FUNCTION_BLOCK Reset_Driver_Fault_AC_Drives_DUT

VAR_IN_OUT
    SD_SMD_IO: DUT_AMCI_Stepper;
END_VAR	

VAR_INPUT
			
END_VAR

VAR_OUTPUT

END_VAR

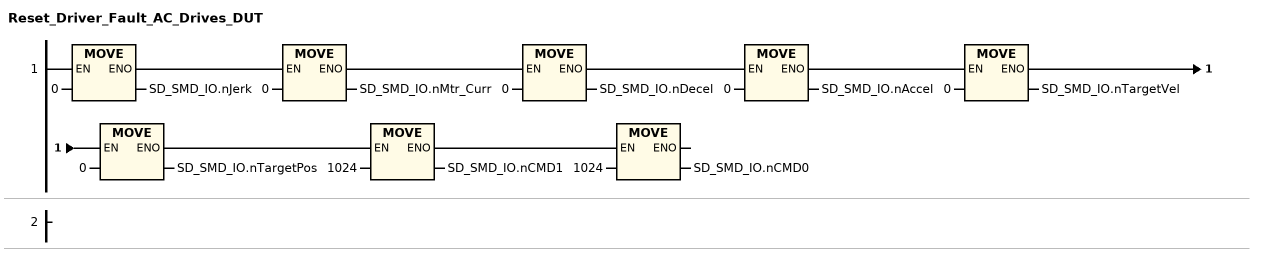
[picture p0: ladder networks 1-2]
// NETWORK 1
SD_SMD_IO.nJerk := 0;
SD_SMD_IO.nMtr_Curr := 0;
SD_SMD_IO.nDecel := 0;
SD_SMD_IO.nAccel := 0;
SD_SMD_IO.nTargetVel := 0;
SD_SMD_IO.nTargetPos := 0;
SD_SMD_IO.nCMD1 := 1024;
SD_SMD_IO.nCMD0 := 1024;

// NETWORK 2

END_FUNCTION_BLOCK
